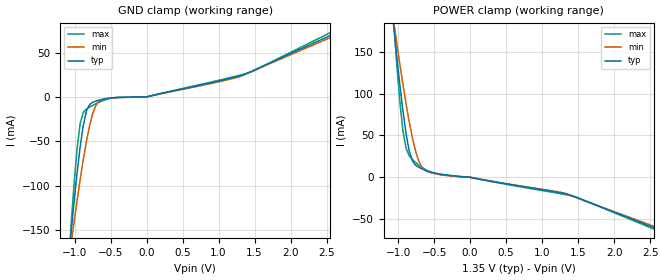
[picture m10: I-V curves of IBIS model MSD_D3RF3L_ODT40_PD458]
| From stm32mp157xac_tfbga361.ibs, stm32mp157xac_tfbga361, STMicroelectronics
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[Model] MSD_D3RF3L_ODT40_PD458
Model_type   Input
C_comp 2.330pF   2.291pF   2.382pF
Vinh = 810.000mV
Vinl = 540.000mV
[Temperature Range]   25.000   125.000   -40.000
[Voltage Range]   1.350V   1.283V   1.450V
[GND Clamp Reference]   0.00V   0.00V   0.00V
[POWER Clamp Reference]   1.350V   1.283V   1.450V
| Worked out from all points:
|   GND clamp passes 1 mA (typ) near -0.47 V on its own axis
|   POWER clamp passes 1 mA (typ) near -0.15 V on its own axis
[GND Clamp]
-1.318V   -415.4mA   -341.4mA   -533.5mA
-1.055V   -159.3mA   -170.5mA   -153.4mA
-1.011V   -121.7mA   -143.7mA   -102.7mA
-966.7mV  -87.2mA    -118mA     -59.85mA
-922.7mV  -56.77mA   -93.49mA   -30.25mA
-878.8mV  -32.1mA    -70.78mA   -17.59mA
-834.9mV  -15.96mA   -50.17mA   -13.63mA
-747mV    -6.03mA    -18.57mA   -9.49mA
-615.1mV  -2.85mA    -2.852mA   -4.52mA
200nV     3.87nA     3.647nA    4.059nA
1.45V     28.54mA    28.18mA    27.96mA
2.68V     73.9mA     71.3mA     77.58mA
[Power Clamp]
-1.33V    440.9mA    363.5mA    565.9mA
-1.067V   185mA      190.2mA    192.4mA
-1.023V   147.7mA    163mA      140.1mA
-978.8mV  112.9mA    136.7mA    93.38mA
-934.9mV  80.78mA    111.7mA    56.6mA
-890.9mV  52.9mA     88.3mA     35.17mA
-847mV    31.77mA    66.79mA    25.86mA
-759.1mV  14.63mA    31.55mA    17.7mA
-671.2mV  10.11mA    12.2mA     11.83mA
-583.3mV  7.179mA    6.41mA     7.369mA
1.438V    -22.9mA    -23.29mA   -22.63mA
2.668V    -64.06mA   -62.26mA   -66.08mA
